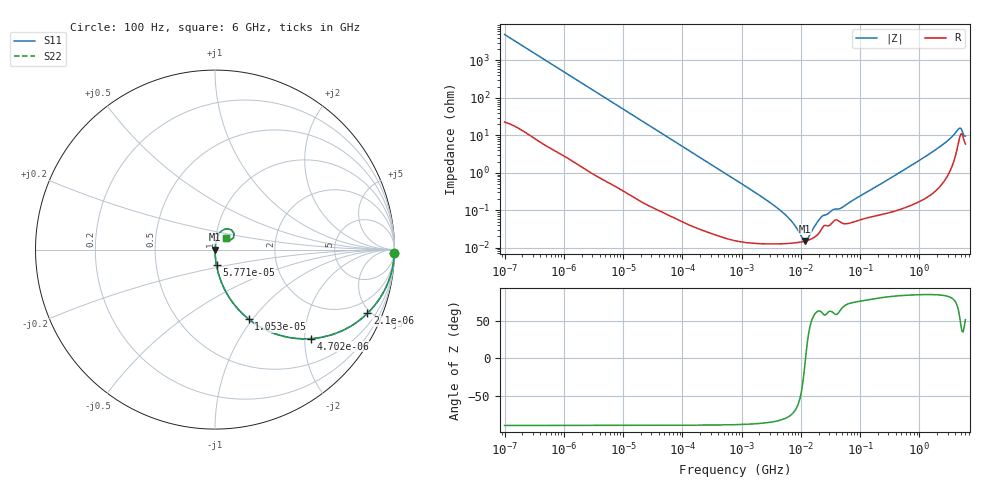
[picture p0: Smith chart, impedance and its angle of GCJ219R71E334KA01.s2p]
!Murata Part Number: GCJ219R71E334KA01
!These Parameters are Measured in Series Mode Connection
!Data Generated on Mar 13, 2026
!  o--ll--o
!Port1  Port2
!  o------o
!Operation Temp=25[degC], DC Bias Voltage=0[V]
!Freq. Start=100[Hz] Stop=6[GHz] 401[Steps]
# Hz S RI R 50
!Freq.(Hz) S11(Real) S11(Imag) S21(Real) S21(Imag) S12(Real) S12(Imag) S22(Real) S22(Imag)
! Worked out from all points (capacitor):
!   401 points, 100 Hz to 6 GHz, reference 50 ohm
!   read as one part in series: C = 321 nF near 109 Hz
!   lowest |Z| = 15 mohm at 11.89 MHz (marker M1)
!   series resonance near 12.02 MHz, so ESL is about 550 pH
!   S11 on the Smith chart (normalised r, x): 100 Hz: open; 2.1 kHz: 1.03, -4.77; 4.702 kHz: 1.01, -2.14; 10.53 kHz: 1.01, -0.96; 57.71 kHz: 1.00, -0.18; 6 GHz: 1.12, +0.15
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100  0.9995 -0.0202  0.000499 0.0202  0.000499 0.0202  0.9995 -0.0202
548  0.9875 -0.1084  0.0125 0.1084  0.0125 0.1084  0.9875 -0.1084
2008  0.8603 -0.3439  0.1397 0.3439  0.1397 0.3439  0.8603 -0.3439
2100  0.8493 -0.3549  0.1507 0.3549  0.1507 0.3549  0.8493 -0.3549
4702  0.5331 -0.4959  0.4669 0.4959  0.4669 0.4959  0.5331 -0.4959
10527  0.1883 -0.3877  0.8117 0.3877  0.8117 0.3877  0.1883 -0.3877
18841  0.0686 -0.2494  0.9314 0.2494  0.9314 0.2494  0.0686 -0.2494
40335  0.0165 -0.1235  0.9835 0.1235  0.9835 0.1235  0.0165 -0.1235
57709  0.00841 -0.0872  0.9916 0.0872  0.9916 0.0872  0.00841 -0.0872
774597  0.000197 -0.00661  0.9998 0.00661  0.9998 0.00661  0.000197 -0.00661
4856642  0.000128 -0.000889  0.9999 0.000889  0.9999 0.000889  0.000128 -0.000889
7266822  0.000132 -0.000452  0.9999 0.000452  0.9999 0.000452  0.000132 -0.000452
1.087309e7  0.000145 -8.68e-05  0.9999 8.68e-05  0.9999 8.68e-05  0.000145 -8.68e-05
1.189169e7  0.00015 -8.9e-06  0.9998 8.9e-06  0.9998 8.9e-06  0.00015 -8.9e-06
1.300572e7  0.000157 6.95e-05  0.9998 -6.95e-05  0.9998 -6.95e-05  0.000157 6.95e-05
1.555665e7  0.000175 0.000231  0.9998 -0.000231  0.9998 -0.000231  0.000175 0.000231
2.327686e7  0.000346 0.000616  0.9997 -0.000616  0.9997 -0.000616  0.000346 0.000616
4.983056e7  0.000452 0.0011  0.9995 -0.0011  0.9995 -0.0011  0.000452 0.0011
3.124326e8  0.000907 0.00685  0.9991 -0.00685  0.9991 -0.00685  0.000907 0.00685
1.95892e9  0.00527 0.0426  0.9947 -0.0426  0.9947 -0.0426  0.00527 0.0426
4.586474e9  0.0742 0.1156  0.9258 -0.1156  0.9258 -0.1156  0.0742 0.1156
6e9  0.0601 0.0666  0.9399 -0.0666  0.9399 -0.0666  0.0601 0.0666
